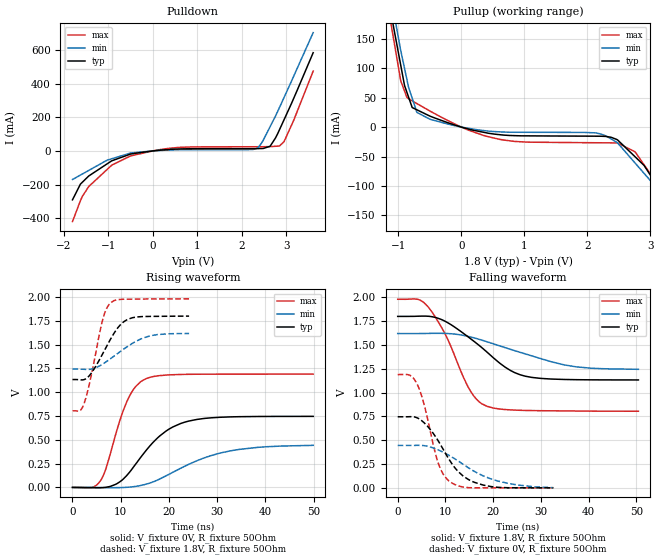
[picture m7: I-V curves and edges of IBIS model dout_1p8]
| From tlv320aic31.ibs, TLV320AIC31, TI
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|   dout_1p8 Model
[Model]   dout_1p8
Model_type   Output
Polarity   Non-Inverting
Vmeas = 0.9
Vref = 0.9
Cref = 10pF
Rref = 50
|   typ   min   max
|   (nom PVT)   (fast PVT)   (slow PVT)
|C_comp from frequency sweep method (F=25MHz)
|C_comp   1.606e-11   1.373e-11   1.680e-11
|ON state : BUFFER OUTPUT TURNED HIGH
|C_comp   1.606e-11   1.373e-11   1.680e-11
|OFF state: BUFFER OUTPUT TURNED LOW
|C_comp   1.381e-11   1.172e-11   1.543e-11
|C_comp from LC tank measurement(L=1nH)
|Resonant Frequency(Hz)   2.010e+09   2.020e+09   1.990e+09
C_comp   6.276e-12   6.214e-12   6.403e-12
|ON state : BUFFER OUTPUT TURNED HIGH
|Resonant Frequency(Hz)   2.010e+09   2.020e+09   1.990e+09
|C_comp   6.276e-12   6.214e-12   6.403e-12
|OFF state: BUFFER OUTPUT TURNED LOW
|Resonant Frequency(Hz)   2.070e+09   2.070e+09   2.070e+09
|C_comp   5.917e-12   5.917e-12   5.917e-12
| Where nom  PVT is Nominal Process, 1.8V, 26C
|   Fast PVT is Strong Process,  1.98V, -40C
|   Slow PVT is Weak Process,   1.62V, 86C
[Voltage Range]   1.8   1.62   1.98
|Ambient Temperature   25   85   -40
|Junction Temperature
[Temperature Range]   26   86   -40
[Pullup Reference]   1.8   1.62   1.98
[Pulldown Reference]   0   0   0
[Power Clamp Reference]   1.8   1.62   1.98
[GND Clamp Reference]   0   0   0
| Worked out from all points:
|   slope of the pulldown table from 0 to 0.27 V, typ, clamps not added: 39.1 ohm
|   slope of the pullup table from 0 to 0.27 V, typ, clamps not added: 38.1 ohm
|   falling waveform, V_fixture 1.8V, R_fixture 50Ohm: 20-80 % time 9.99ns typ, 14.5ns min, 6.5ns max; typ from 1.8 V to 1.13 V
|   rising waveform, V_fixture 0V, R_fixture 50Ohm: 20-80 % time 7.89ns typ, 12ns min, 4.57ns max; typ from 0 V to 0.746 V
|   rising waveform, V_fixture 1.8V, R_fixture 50Ohm: 20-80 % time 4.48ns typ, 6.55ns min, 2.89ns max; typ from 1.13 V to 1.8 V
|   falling waveform, V_fixture 0V, R_fixture 50Ohm: 20-80 % time 6.07ns typ, 9.56ns min, 3.55ns max; typ from 0.746 V to 0 V
[Pulldown]
|   Voltage   I(typ)   I(min)   I(max)
-1.8V     -289.9mA   -169.2mA   -418.8mA
-1.624V   -197.6mA   -143.2mA   -296.2mA
-1.434V   -148.2mA   -115.2mA   -210.6mA
-916.7mV  -58.22mA   -46.08mA   -83.68mA
-495mV    -18.15mA   -12.21mA   -29.2mA
568.3mV   11.57mA    6.86mA     20.7mA
2.336V    13.94mA    15.71mA    25.01mA
2.461V    14.57mA    55.25mA    25.09mA
2.633V    27.78mA    143.9mA    25.8mA
2.843V    125.6mA    257.7mA    29.37mA
2.946V    185.2mA    317.3mA    55.63mA
3.6V      583.1mA    702.3mA    474mA
[Pullup]
|   Voltage   I(typ)   I(min)   I(max)
-1.8V     624.8mA    624.7mA    653.2mA
-1.195V   238.8mA    268mA      225.6mA
-962.3mV  105.8mA    130.6mA    79.41mA
-863.3mV  59.12mA    80.87mA    50.46mA
-704.7mV  29.31mA    24.92mA    39.94mA
-494.1mV  18.41mA    13.17mA    26.99mA
653.4mV   -13.45mA   -8.357mA   -21.73mA
2.479V    -21.82mA   -26.87mA   -27.05mA
2.756V    -50.43mA   -61.05mA   -42mA
3.355V    -145mA     -134.8mA   -156.5mA
3.453V    -177.9mA   -146.9mA   -179.4mA
3.6V      -254.1mA   -165mA     -246.1mA
[Ramp]
R_load = 50
|   typ   min   max
dV/dt_r   0.447678/7.8807e-09   0.266805/1.21122e-08   0.713753/4.54886e-09
dV/dt_f   0.400381/9.98955e-09   0.226416/1.45738e-08   0.705276/6.48785e-09
[Falling Waveform]
V_fixture = 1.8V
V_fixture_min = 1.62V
V_fixture_max = 1.98V
R_fixture = 50Ohm
|   Time   V(typ)   V(min)   V(max)
0s        1.8V       1.62V      1.98V
4.185ns   1.802V     1.62V      1.98V
6.42ns    1.802V     1.622V     1.897V
10.04ns   1.746V     1.621V     1.605V
15.13ns   1.571V     1.586V     1.026V
18.69ns   1.426V     1.534V     856.6mV
22.53ns   1.266V     1.472V     822.1mV
26.81ns   1.171V     1.405V     812.6mV
37.43ns   1.136V     1.27V      806.7mV
50.41ns   1.133V     1.245V     804.6mV
[Rising Waveform]
V_fixture = 0V
V_fixture_min = 0V
V_fixture_max = 0V
R_fixture = 50Ohm
|   Time   V(typ)   V(min)   V(max)
0s        1.07nV     5.284nV    697.7pV
4.005ns   -2.553mV   -393.9uV   -580.4uV
5.78ns    -3.291mV   -1.602mV   69mV
11.33ns   129.8mV    1.28mV     908mV
13.13ns   246.9mV    10.97mV    1.061V
15.36ns   394.4mV    35.37mV    1.144V
20.08ns   614.4mV    139.8mV    1.182V
25.69ns   713mV      278.3mV    1.189V
34.5ns    742.6mV    398.9mV    1.189V
49.89ns   746mV      441.7mV    1.19V
[Rising Waveform]
V_fixture = 1.8V
V_fixture_min = 1.62V
V_fixture_max = 1.98V
R_fixture = 50Ohm
|   Time   V(typ)   V(min)   V(max)
0s        1.133V     1.242V     804.5mV
1.51ns    1.131V     1.242V     804.1mV
2.37ns    1.132V     1.24V      876.7mV
3.6ns     1.18V      1.24V      1.108V
6.06ns    1.385V     1.289V     1.722V
7.835ns   1.553V     1.35V      1.936V
9.935ns   1.708V     1.428V     1.974V
12.4ns    1.781V     1.512V     1.977V
16.45ns   1.796V     1.595V     1.979V
24.17ns   1.799V     1.616V     1.98V
[Falling Waveform]
V_fixture = 0V
V_fixture_min = 0V
V_fixture_max = 0V
R_fixture = 50Ohm
|   Time   V(typ)   V(min)   V(max)
0s        746.1mV    445.3mV    1.19V
2.5ns     746.9mV    445.2mV    1.184V
3.985ns   737mV      446.1mV    1.098V
5.46ns    686.8mV    443.4mV    887.8mV
8.56ns    487.1mV    396.4mV    249.7mV
10.75ns   299.4mV    340.8mV    71.6mV
13.62ns   127.4mV    250mV      9.284mV
17.85ns   29.94mV    126.9mV    480uV
25.03ns   694.8uV    30.63mV    43.91uV
32.61ns   140.6uV    2.066mV    3.274uV
